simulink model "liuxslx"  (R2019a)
settings: configuration reference "configurationSettings" (kept in a data dictionary, not in this file)
libraries: liulib x1

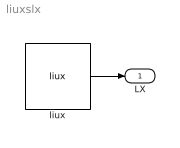
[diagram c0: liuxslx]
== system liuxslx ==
  liux : liulib/liux  SystemSampleTime=-1
  LX : Outport  OutDataTypeStr=Bus: LXbus
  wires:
  liux/1 -> LX/1
